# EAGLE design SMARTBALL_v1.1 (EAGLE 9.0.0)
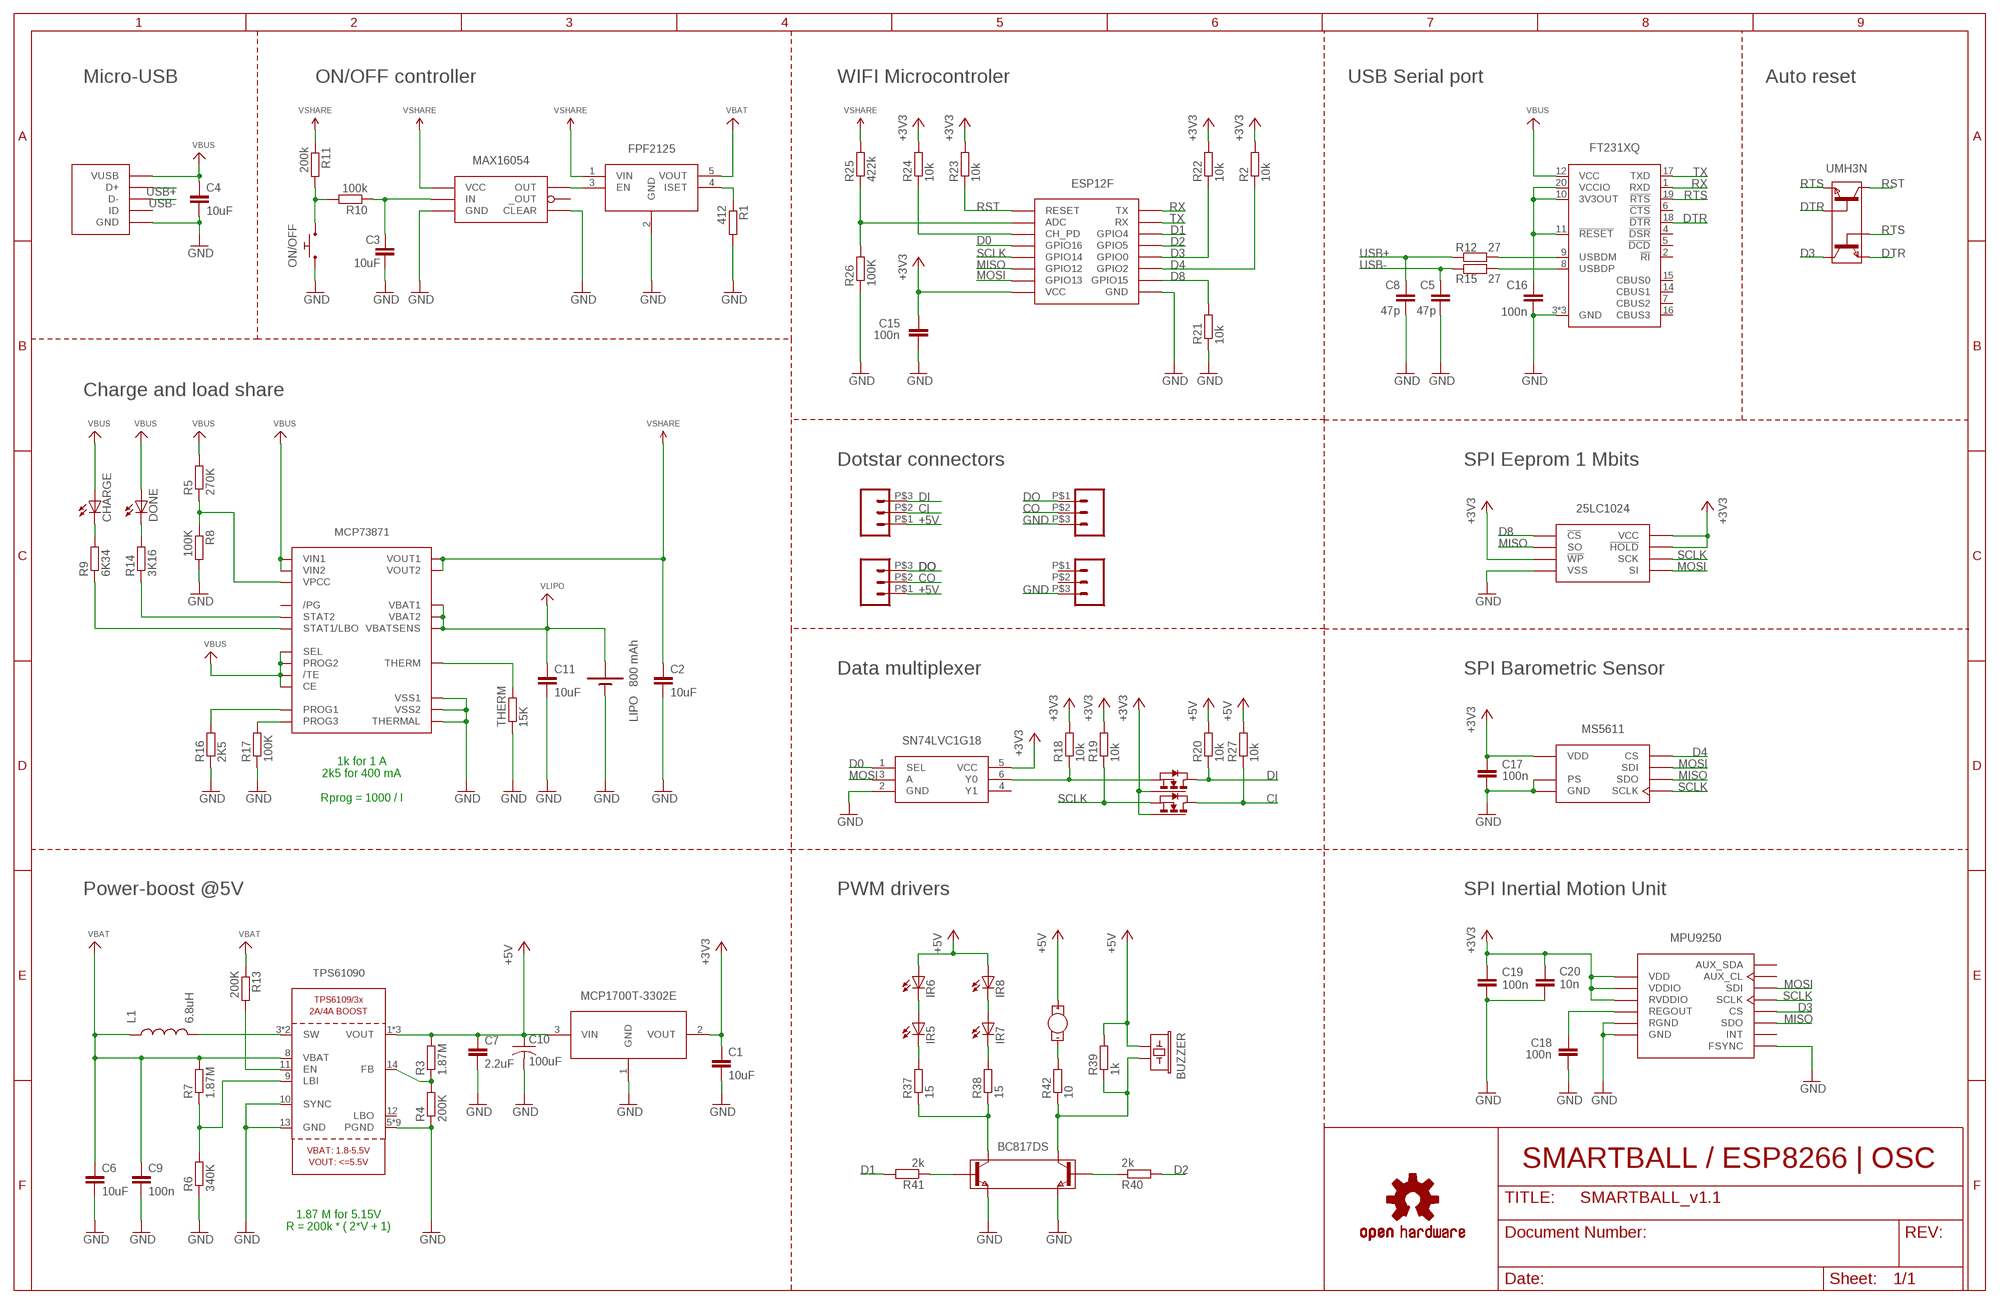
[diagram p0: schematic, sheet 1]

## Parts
BC817DS  BC817DS  [SOT457R_PHILIPS]
BUZZER  BUZZER_PKMCS0909E4000-R1  [BUZZER_PKMCS0909E4000-R1]
C1  10uF  C-EUC0603K  [C0603K]
C2  10uF  C-EUC0603K  [C0603K]
C3  10uF  C-EUC0603K  [C0603K]
C4  10uF  C-EUC0603K  [C0603K]
C5  47p  C-EUC0603K  [C0603K]
C6  10uF  C-EUC0603K  [C0603K]
C7  2.2uF  C-EUC0603K  [C0603K]
C8  47p  C-EUC0603K  [C0603K]
C9  100n  C-EUC0603K  [C0603K]
C10  100uF  C-USC1210  [C1210]
C11  10uF  C-EUC0603K  [C0603K]
C15  100n  C-EUC0603K  [C0603K]
C16  100n  C-EUC0603K  [C0603K]
C17  100n  C-EUC0603K  [C0603K]
C18  100n  C-EUC0603K  [C0603K]
C19  100n  C-EUC0603K  [C0603K]
C20  10n  C-EUC0603K  [C0603K]
CHARGE  KINGBRIGHT_16X08  [KINGBRIGHT_16X08]
DONE  KINGBRIGHT_16X08  [KINGBRIGHT_16X08]
ESP12F  ESP12  [ESP12]
FT231XQ  FT231X  [QFN20]
IR5  LED-SFH4050  [SFH4050]
IR6  LED-SFH4050  [SFH4050]
IR7  LED-SFH4050  [SFH4050]
IR8  LED-SFH4050  [SFH4050]
L1  6.8uH  ASPIAIG-S4035  [ASPIAIG-S4035]
LIPO  BATTERY_CONNECTOR  [MOTOR_CONNECTOR]
LOGO1  OSHW-LOGOL  [OSHW-LOGO-L]
MCP73871  MCP73871  [QFN20_4MM]
MOTOR  MOTOR_CONNECTOR  [MOTOR_CONNECTOR]
ON/OFF  B3U-3000P-B  [B3U-3000P-B]
R1  412  R-EU_R0402  [R0402]
R2  10k  R-EU_R0402  [R0402]
R3  1.87M  R-EU_R0402  [R0402]
R4  200K  R-EU_R0402  [R0402]
R5  270K  R-EU_R0402  [R0402]
R6  340K  R-EU_R0402  [R0402]
R7  1.87M  R-EU_R0402  [R0402]
R8  100K  R-EU_R0402  [R0402]
R9  6K34  R-EU_R0402  [R0402]
R10  100k  R-EU_R0402  [R0402]
R11  200k  R-EU_R0402  [R0402]
R12  27  R-EU_R0402  [R0402]
R13  200K  R-EU_R0402  [R0402]
R14  3K16  R-EU_R0402  [R0402]
R15  27  R-EU_R0402  [R0402]
R16  2K5  R-EU_R0402  [R0402]
R17  100K  R-EU_R0402  [R0402]
R18  10k  R-EU_R0402  [R0402]
R19  10k  R-EU_R0402  [R0402]
R20  10k  R-EU_R0402  [R0402]
R21  10k  R-EU_R0402  [R0402]
R22  10k  R-EU_R0402  [R0402]
R23  10k  R-EU_R0402  [R0402]
R24  10k  R-EU_R0402  [R0402]
R25  422k  R-EU_R0402  [R0402]
R26  100K  R-EU_R0402  [R0402]
R27  10k  R-EU_R0402  [R0402]
R37  15  R-EU_R0402  [R0402]
R38  15  R-EU_R0402  [R0402]
R39  1k  R-EU_R0402  [R0402]
R40  2k  R-EU_R0402  [R0402]
R41  2k  R-EU_R0402  [R0402]
R42  10  R-EU_R0402  [R0402]
THERM  15K  R-EU_R0402  [R0402]
TPS61090  TPS61090RSAR  VREG_TPS6103X  [PVQFN-16]
U$1  MOLEX-USB  [MOLEX-USB]
U$2  FPF2125  [SOT23-5]
U$3  MCP1700T  [SOT23-3]
U$5  CONN_03_SMD  [CONN03_SMD]
U$6  CONN_03_SMD  [CONN03_SMD]
U$12  MAX16054  [TSOT23-6]
U$14  CONN_03_SMD  [CONN03_SMD]
U$15  CONN_03_SMD  [CONN03_SMD]
U$16  25LC1024DFN-S  [DFN-S]
U$17  MS5611  [MS5611-QFN]
U$20  SN74LVC1G18  [DCK_R-PDSO-G6]
U$21  MPU-9250QFN24G  [QFN24G-0.4-3X3MM]
U$22  2N7002PS  [SOT363_PHILIPS]
UMH3N  UMH3N  [SOT363_PHILIPS]

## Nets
+3V3 [+3v3]: C1.1 C15.1 C17.1 C19.1 C20.2 ESP12F.VCC R2.2 R18.2 R19.2 R22.2 R23.2 R24.2 U$3.2(VOUT) U$16.3(!WP) U$16.7(!HOLD) U$16.8(VCC) U$17.P$1(VDD) U$20.5(VCC) U$21.1(RVDDIO) U$21.8(VDDIO) U$21.13(VDD) U$22.2(G1) U$22.5(G2)
+5V [power]: BUZZER.P$1 C7.1 C10.1 IR6.P$1(A) IR8.P$1(A) MOTOR.+ R3.2 R20.2 R27.2 R39.2 TPS61090.1(VOUT) TPS61090.15(VOUT) TPS61090.16(VOUT) U$3.3(VIN) U$5.P$1 U$15.P$1
CI: R27.1 U$5.P$2 U$22.3(D2)
CO: U$6.P$2 U$15.P$2
D0: ESP12F.GPIO16 U$20.1(SEL)
D1: ESP12F.GPIO4 R41.2
D2: ESP12F.GPIO5 R40.2
D3: ESP12F.GPIO0 R22.1 U$21.22(CS) UMH3N.3(C2)
D4: ESP12F.GPIO2 R2.1 U$17.P$4(CS) U$17.P$5(CS)
D8: ESP12F.GPIO15 R21.2 U$16.1(!CS)
DI: R20.1 U$5.P$3 U$22.6(D1)
DO: U$6.P$1 U$15.P$3
DTR: FT231XQ.18(!DTR) UMH3N.2(B1) UMH3N.4(E2)
EN1: ESP12F.CH_PD R24.1
ENABLE: R13.2 TPS61090.11(EN)
GND [power]: BC817DS.1(E1) BC817DS.4(E2) C1.2 C2.2 C3.2 C4.2 C5.2 C6.2 C7.2 C8.2 C9.2 C10.2 C11.2 C15.2 C16.2 C17.2 C18.2 C19.2 C20.1 ESP12F.GND FT231XQ.3(GND) FT231XQ.13(GND) FT231XQ.EXP(GND) LIPO.- MCP73871.P$10(VSS1) MCP73871.P$11(VSS2) MCP73871.P$21(THERMAL) ON/OFF.P$1 R1.2 R4.1 R6.1 R8.2 R16.1 R17.1 R21.1 R26.1 THERM.1 TPS61090.5(PGND) TPS61090.6(PGND) TPS61090.7(PGND) TPS61090.10(SYNC) TPS61090.13(GND) TPS61090.P$18(PGND) TPS61090.P$19(PGND) TPS61090.P$20(PGND) TPS61090.P$21(PGND) TPS61090.P$22(PGND) TPS61090.THERMAL(PGND) U$1.GND U$1.P$1(GND) U$1.P$11(GND) U$1.SHELL1(GND) U$1.SHELL2(GND) U$1.SHELL5(GND) U$1.SHELL6(GND) U$2.2(GND) U$3.1(GND) U$6.P$3 U$12.CLEAR U$12.GND U$14.P$3 U$16.4(VSS) U$17.P$2(PS) U$17.P$3(GND) U$20.2(GND) U$21.11(FSYNC) U$21.18(GND) U$21.20(RGND)
MISO: ESP12F.GPIO12 U$16.2(SO) U$17.P$6(SDO) U$21.9(SDO)
MOSI: ESP12F.GPIO13 U$16.5(SI) U$17.P$7(SDI) U$20.3(A) U$21.24(SDI)
N$1: U$2.3(EN) U$12.OUT
N$2: R1.1 U$2.4(ISET)
N$3: MCP73871.P$2(VPCC) R5.1 R8.1
N$4: MCP73871.P$13(PROG1) R16.2
N$5: FT231XQ.9(USBDM) R12.2
N$6: FT231XQ.8(USBDP) R15.2
N$8: ON/OFF.P$2 R10.2 R11.2
N$9: C3.1 R10.1 U$12.IN
N$11: R18.1 U$20.6(Y0) U$22.1(S1)
N$12: ESP12F.ADC R25.1 R26.2
N$17: L1.P$2 TPS61090.3(SW) TPS61090.4(SW)
N$18: R6.2 R7.1 TPS61090.9(LBI)
N$21: R3.1 R4.2 TPS61090.14(FB)
N$22: MCP73871.P$7(STAT2) R14.1
N$23: MCP73871.P$8(STAT1/LBO) R9.1
N$25: MCP73871.P$5(THERM) THERM.2
N$26: DONE.CATHODE(C) R14.2
N$27: CHARGE.CATHODE(C) R9.2
N$28: MCP73871.P$12(PROG3) R17.2
N$55: IR5.P$2(C) R37.2
N$56: IR5.P$1(A) IR6.P$2(C)
N$57: BC817DS.3(C2) R37.1 R38.1
N$58: IR7.P$2(C) R38.2
N$59: IR7.P$1(A) IR8.P$2(C)
N$60: BC817DS.6(C1) BUZZER.P$2 R39.1 R42.1
N$61: MOTOR.- R42.2
N$62: BC817DS.5(B2) R41.1
N$63: BC817DS.2(B1) R40.1
REGOUT1: C18.1 U$21.10(REGOUT)
RST: ESP12F.RESET R23.1 UMH3N.6(C1)
RTS: FT231XQ.19(!RTS) UMH3N.1(E1) UMH3N.5(B2)
RX: ESP12F.TX FT231XQ.1(RXD)
SCLK: ESP12F.GPIO14 R19.1 U$16.6(SCK) U$17.P$8(SCLK) U$21.23(SCLK) U$22.4(S2)
TX: ESP12F.RX FT231XQ.17(TXD)
USB+: C8.1 R12.1 U$1.D+
USB-: C5.1 R15.1 U$1.D-
VBAT [power]: C6.1 C9.1 L1.P$1 R7.2 R13.1 TPS61090.8(VBAT) U$2.5(VOUT)
VBUS [power]: C4.1 CHARGE.ANODE(A) DONE.ANODE(A) FT231XQ.12(VCC) MCP73871.P$3(SEL) MCP73871.P$4(PROG2) MCP73871.P$9(/TE) MCP73871.P$17(CE) MCP73871.P$18(VIN1) MCP73871.P$19(VIN2) R5.2 U$1.VUSB
VCCIO1: C16.1 FT231XQ.10(3V3OUT) FT231XQ.11(!RESET) FT231XQ.20(VCCIO)
VLIPO: C11.1 LIPO.+ MCP73871.P$14(VBAT1) MCP73871.P$15(VBAT2) MCP73871.P$16(VBATSENS)
VSHARE [power]: C2.1 MCP73871.P$1(VOUT1) MCP73871.P$20(VOUT2) R11.1 R25.2 U$2.1(VIN) U$12.VCC
Unconnected: FT231XQ.2(!RI) FT231XQ.4(!DSR) FT231XQ.5(!DCD) FT231XQ.6(!CTS) FT231XQ.7(CBUS2) FT231XQ.14(CBUS1) FT231XQ.15(CBUS0) FT231XQ.16(CBUS3) MCP73871.P$6(/PG) TPS61090.12(LBO) U$1.ID U$12._OUT U$14.P$1 U$14.P$2 U$20.4(Y1) U$21.7(AUX_CL) U$21.12(INT) U$21.21(AUX_SDA)

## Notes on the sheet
- Micro-USB | ON/OFF controller | WIFI Microcontroler | USB Serial port | Auto reset
- FPF2125
- MAX16054
- Charge and load share
- Dotstar connectors | SPI Eeprom 1 Mbits
- Data multiplexer | SPI Barometric Sensor
- 800 mAh
- SN74LVC1G18
- 1k for 1 A
  2k5 for 400 mA
  
  Rprog = 1000 / I
- Power-boost @5V | PWM drivers | SPI Inertial Motion Unit
- MCP1700T-3302E
- SMARTBALL / ESP8266 | OSC
- 1.87 M for 5.15V
  R = 200k * ( 2*V + 1)

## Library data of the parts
BC817DS = Smartball:BC817DS
BUZZER = Smartball:BUZZER_PKMCS0909E4000-R1
C1-C9 C11 C15-C20 = rcl:C-EU: CAPACITOR, European symbol; SPICEPREFIX: C
C10 = rcl:C-US: CAPACITOR, American symbol
CHARGE DONE = Smartball:KINGBRIGHT_16X08
ESP12F = esp8266modules:ESP12: ESP8266 Wifi module 12
FT231XQ = Smartball:FT231X
IR5-IR8 = Smartball:LED-SFH4050: 850 nm High Power IR Led from OSRAM
L1 = Smartball:ASPIAIG-S4035
LIPO = Smartball:BATTERY_CONNECTOR
LOGO1 = SparkFun-Aesthetics:OSHW-LOGO: Open-Source Hardware (OSHW) Logo
MCP73871 = microbuilder:MCP73871: MCP73871 Lithium Polymer Battery Charger Digikey: MCP73871-2CCI/ML-ND
MOTOR = Smartball:MOTOR_CONNECTOR
ON/OFF = Smartball:B3U-3000P-B
R1-R27 R37-R42 THERM = rcl:R-EU_: RESISTOR, European symbol; SPICEPREFIX: R
TPS61090 = microbuilder:VREG_TPS6103X: TPS6103x 4A Boost - 1.8-5.5V Input, Adjustable Output to 5.5V
U$1 = Smartball:MOLEX-USB
U$2 = Smartball:FPF2125
U$3 = Smartball:MCP1700T
U$5 U$6 U$14 U$15 = Smartball:CONN_03_SMD
U$12 = Smartball:MAX16054
U$16 = Smartball:25LC1024: Microship 25LC1024 1Mbit SPI EEPROM
U$17 = Smartball:MS5611: MS5611 barometric sensor
U$20 = Smartball:SN74LVC1G18
U$21 = Smartball:MPU-9250: MPU-9250 Invensense IMU Chipset
U$22 = Smartball:2N7002PS
UMH3N = Smartball:UMH3N

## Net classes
0 default: width 0.152 mm
1 power: width 0.254 mm
2 +3v3: width 0.203 mm

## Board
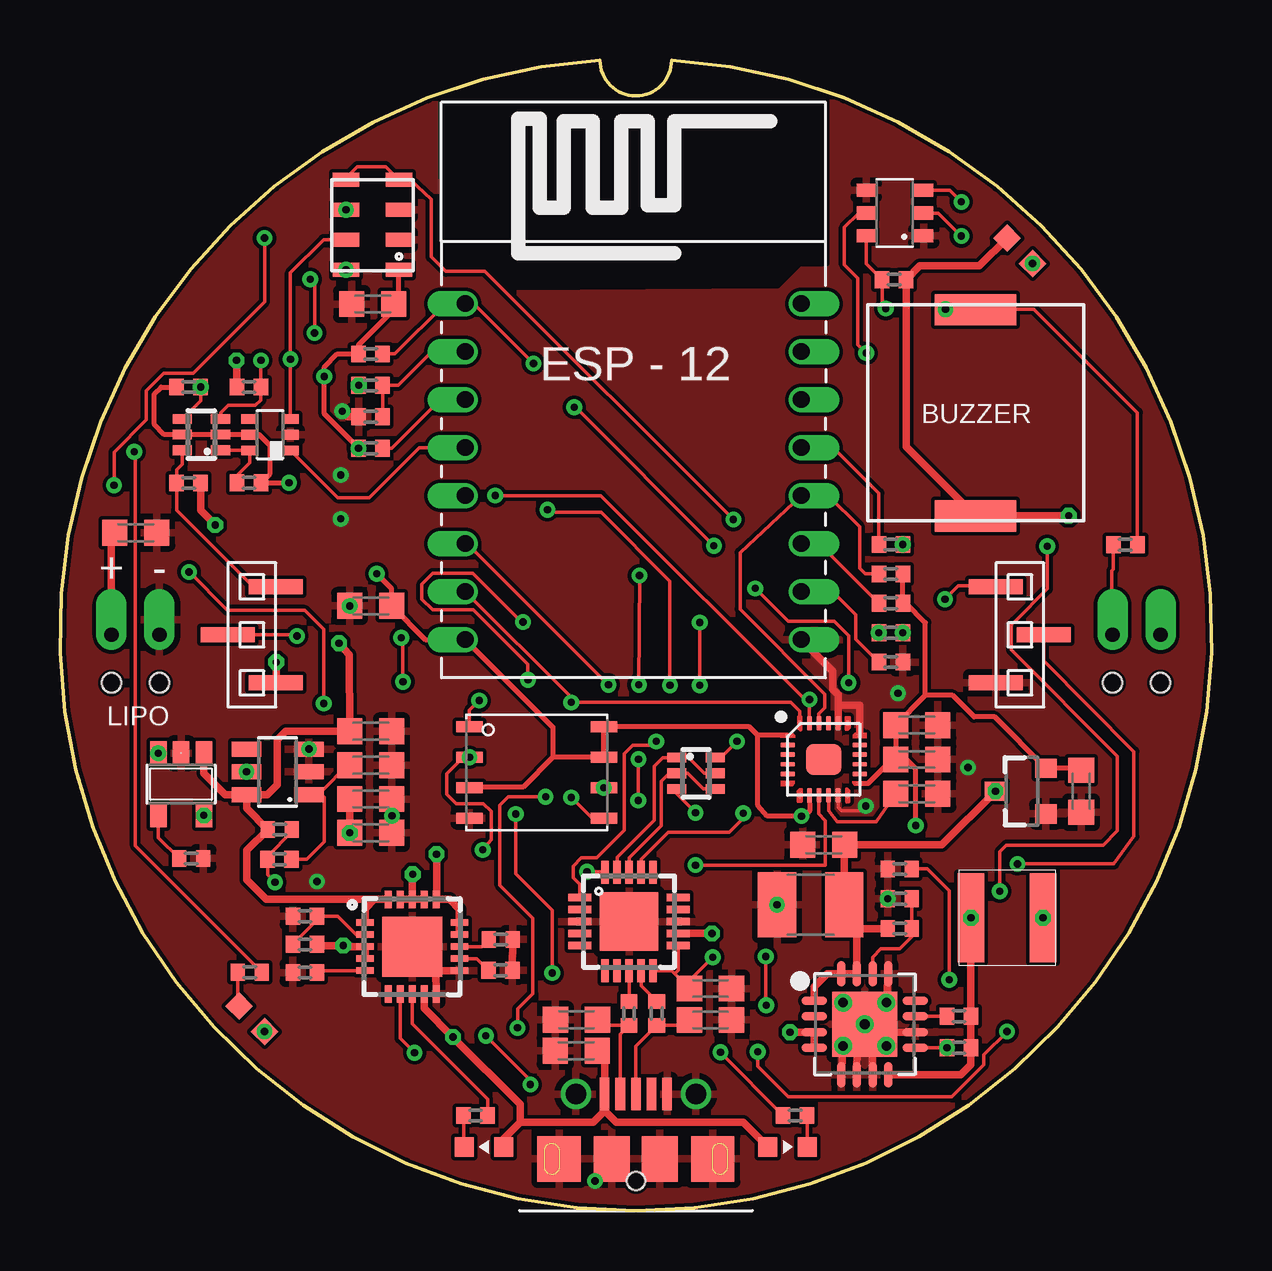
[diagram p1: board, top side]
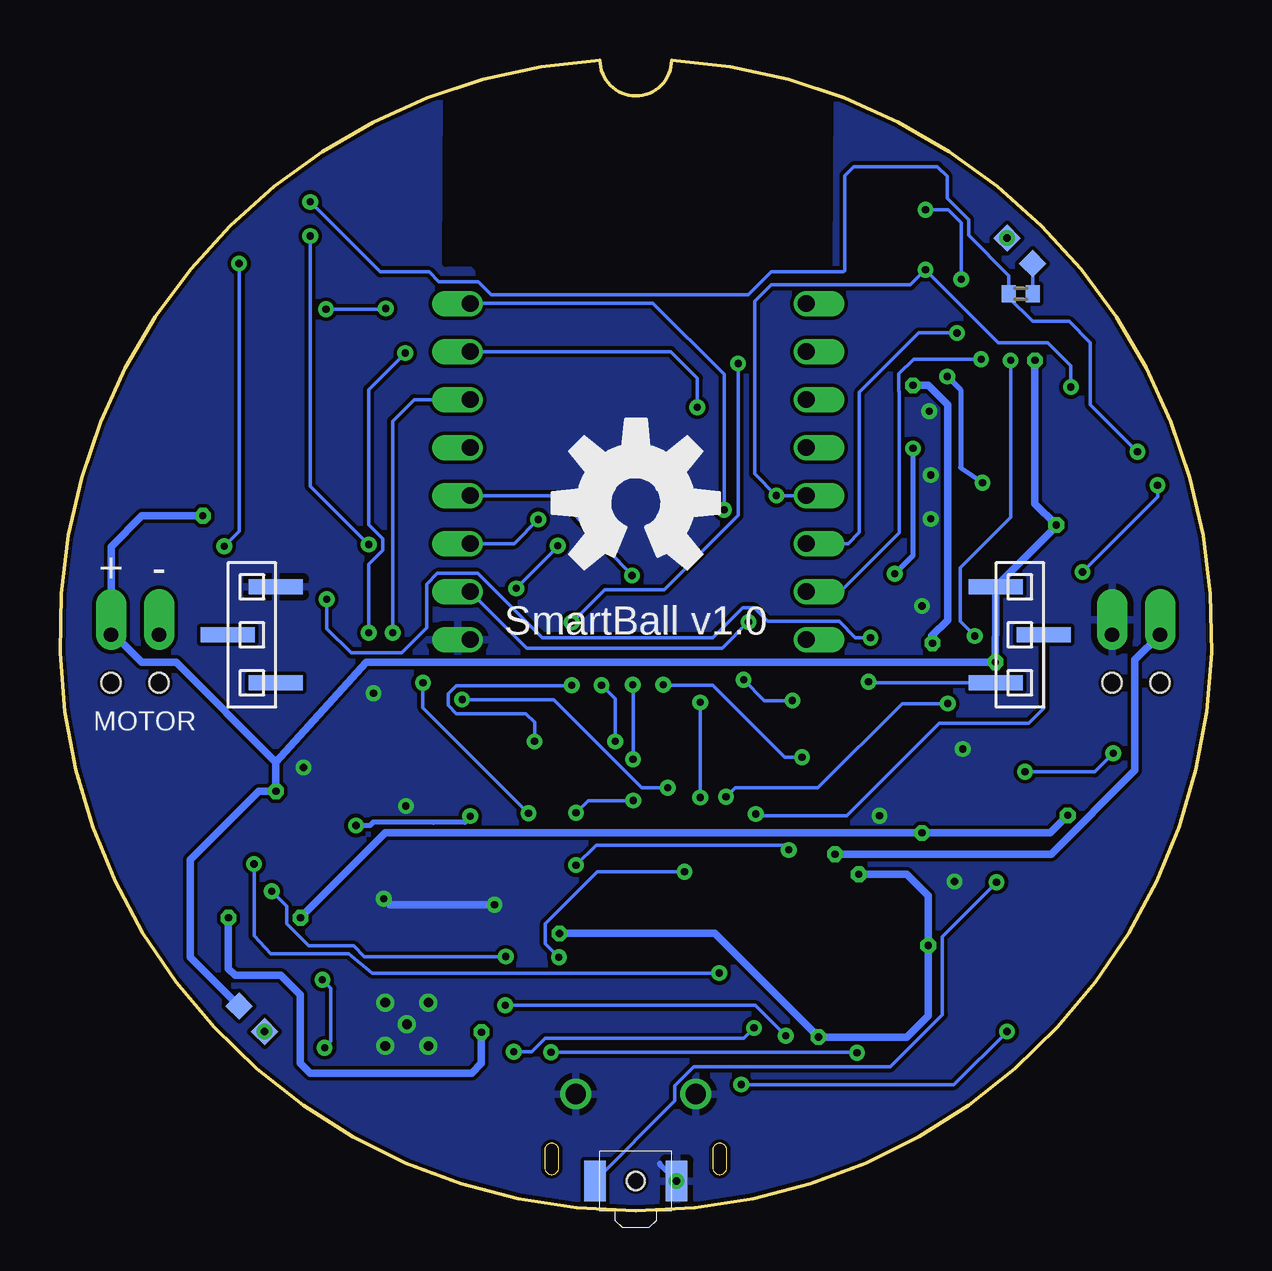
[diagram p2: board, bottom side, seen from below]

Size 47.98 x 47.96 mm. Coordinates in mm from the lower left corner, seen from the top.
Outline: 22.5,47.96 arc353 25.49,47.96 arc-180 22.5,47.96
Copper layers (1*16): Top 0.035mm / dielectric 1.5mm / Bottom 0.035mm
Design rules "PCBWay-LIMIT": minimum track width 4mil, minimum drill 0.3mm, track to track 6mil, track to pad 6mil, pad to pad 6mil, via to via 6mil, smd to smd 6mil, copper to edge 6mil, drill to drill 6mil, minimum pad ring 7mil, minimum via ring 7mil, stop-mask expansion 4mil, vias tented up to drill 25mil, thermal gap 10mil

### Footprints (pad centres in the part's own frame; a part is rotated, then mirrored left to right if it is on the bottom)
SOT457R_PHILIPS = smd 0.55 x 0.8: 1 -0.95,-1.2; 2 0,-1.2; 3 0.95,-1.2; 4 0.95,1.2; 5 0,1.2; 6 -0.95,1.2
BUZZER_PKMCS0909E4000-R1 = smd 1.3 x 3.4: P$1 -4.3,0; P$2 4.3,0
C0603K = smd 1.05 x 1.08: 1 -0.875,0; 2 0.875,0
C1210 = smd 1.6 x 2.7: 1 -1.4,0; 2 1.4,0
KINGBRIGHT_16X08 = smd 0.8 x 0.8: ANODE 0,0; CATHODE 1.65,0
ESP12 = drill 0.7 offset: ADC -7.1,3.8; CH_PD -7.1,1.8; GND 6.9,-8.2; GPIO0 6.9,-2.2; GPIO2 6.9,-4.2; GPIO4 6.9,1.8; GPIO5 6.9,-0.2; GPIO12 -7.1,-4.2; GPIO13 -7.1,-6.2; GPIO14 -7.1,-2.2; GPIO15 6.9,-6.2; GPIO16 -7.1,-0.2; RESET -7.1,5.8; RX 6.9,3.8; TX 6.9,5.8; VCC -7.1,-8.2
QFN20 = smd 0.95 x 0.3: 1 -2.05,1; 2 -2.05,0.5; 3 -2.05,0; 4 -2.05,-0.5; 5 -2.05,-1; 11 2.05,-1; 12 2.05,-0.5; 13 2.05,0; 14 2.05,0.5; 15 2.05,1 | smd 0.3 x 0.95: 6 -1,-2.05; 7 -0.5,-2.05; 8 0,-2.05; 9 0.5,-2.05; 10 1,-2.05; 16 1,2.05; 17 0.5,2.05; 18 0,2.05; 19 -0.5,2.05; 20 -1,2.05 | smd 2.45 x 2.45: EXP 0,0
SFH4050 = smd 0.8 x 0.8: P$1 -0.75,0; P$2 0.75,0
ASPIAIG-S4035 = smd 1.1 x 3.7: P$1 -1.5,0; P$2 1.5,0
MOTOR_CONNECTOR = drill 0.6 pad 1.27 offset: + 0,0; - 2,0 | hole 0.8: 0,-2; 2,-2
QFN20_4MM = smd 0.73 x 0.28: P$1 -1.965,1; P$2 -1.965,0.5; P$3 -1.965,0; P$4 -1.965,-0.5; P$5 -1.965,-1; P$11 1.965,-1; P$12 1.965,-0.5; P$13 1.965,0; P$14 1.965,0.5; P$15 1.965,1 | smd 0.28 x 0.73: P$6 -1,-1.965; P$7 -0.5,-1.965; P$8 0,-1.965; P$9 0.5,-1.965; P$10 1,-1.965; P$16 1,1.965; P$17 0.5,1.965; P$18 0,1.965; P$19 -0.5,1.965; P$20 -1,1.965 | smd 2.5 x 2.5: P$21 0,0
B3U-3000P-B = smd 0.9 x 1.7: P$1 0,0; P$2 3.4,0 | hole 0.75: 1.7,0
R0402 = smd 0.6 x 0.7: 1 -0.5,0; 2 0.5,0
PVQFN-16 = smd 1.05 x 0.35: 1 -2.1,0.975; 2 -2.1,0.325; 3 -2.1,-0.325; 4 -2.1,-0.975; 9 2.1,-0.975; 10 2.1,-0.325; 11 2.1,0.325; 12 2.1,0.975 | smd 0.35 x 1.05: 5 -0.975,-2.1; 6 -0.325,-2.1; 7 0.325,-2.1; 8 0.975,-2.1; 13 0.975,2.1; 14 0.325,2.1; 15 -0.325,2.1; 16 -0.975,2.1 | drill 0.4: P$18 0,0; P$19 -0.9,0.9; P$20 0.9,0.9; P$21 0.9,-0.9; P$22 -0.9,-0.9 | smd 2.7 x 2.7: THERMAL 0,0
MOLEX-USB = smd 0.4 x 1.35: D+ 0,2.7; D- -0.65,2.7; GND 1.3,2.7; ID 0.65,2.7; VUSB -1.3,2.7 | smd 1.8 x 1.9: P$1 -3.2,0; P$11 3.2,0 | drill 0.85: SHELL1 -2.5,2.7; SHELL2 2.5,2.7 | smd 1.5 x 1.9: SHELL5 -1,0; SHELL6 1,0
SOT23-5 = smd 0.69 x 0.99: 1 -0.95,-1.29; 2 0,-1.29; 3 0.95,-1.29; 4 0.95,1.3; 5 -0.95,1.3
SOT23-3 = smd 0.8 x 0.9: 1 -0.95,-1; 2 0.95,-1; 3 0,1.1
CONN03_SMD = smd 0.635 x 2.25: P$1 -2,-1; P$2 0,1; P$3 2,-1
TSOT23-6 = smd 0.62 x 1.22: _OUT 0.95,1.3; CLEAR 0.95,-1.3; GND 0,-1.3; IN -0.95,-1.3; OUT 0,1.3; VCC -0.95,1.3
DFN-S = smd 1.1 x 0.45: 1 -2.8,1.905; 2 -2.8,0.635; 3 -2.8,-0.635; 4 -2.8,-1.905; 5 2.8,-1.905; 6 2.8,-0.635; 7 2.8,0.635; 8 2.8,1.905
MS5611-QFN = smd 1.1 x 0.6: P$1 -2.2,3.75; P$2 -2.2,2.5; P$3 -2.2,1.25; P$4 -2.2,0; P$5 0,0; P$6 0,1.25; P$7 0,2.5; P$8 0,3.75
DCK_R-PDSO-G6 = smd 0.4 x 0.7: 1 -0.65,-0.85; 2 0,-0.85; 3 0.65,-0.85; 4 0.65,0.85; 5 0,0.85; 6 -0.65,0.85
QFN24G-0.4-3X3MM = smd 0.2 x 0.15: 1 -1.5,1; 6 -1.5,-1; 13 1.5,-1; 18 1.5,1 | smd 0.6 x 0.2: 2 -1.5,0.6; 3 -1.5,0.2; 4 -1.5,-0.2; 5 -1.5,-0.6; 14 1.5,-0.6; 15 1.5,-0.2; 16 1.5,0.2; 17 1.5,0.6 | smd 0.15 x 0.2: 7 -1,-1.5; 12 1,-1.5; 19 1,1.5; 24 -1,1.5 | smd 0.2 x 0.6: 8 -0.6,-1.5; 9 -0.2,-1.5; 10 0.2,-1.5; 11 0.6,-1.5; 20 0.6,1.5; 21 0.2,1.5; 22 -0.2,1.5; 23 -0.6,1.5 | smd 1.5 x 1.3: 25 0,0
SOT363_PHILIPS = smd 0.4 x 0.8: 1 -0.65,-0.8; 2 0,-0.8; 3 0.65,-0.8; 4 0.65,0.8; 5 0,0.8; 6 -0.65,0.8

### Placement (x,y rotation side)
BC817DS  34.79,41.58 90 top
BUZZER  38.15,33.26 90 top
C1  42.55,17.49 270 top
C2  12.94,19.99 0 top
C3  12.94,18.58 0 top
C4  21.51,6.67 180 top
C5  21.52,7.97 180 top
C6  12.94,15.76 0 top
C7  31.82,15.26 180 top
C8  27.1,7.96 0 top
C9  12.94,17.17 0 top
C10  31.28,12.76 180 top
C11  3.15,28.26 0 top
C15  12.94,25.21 180 top
C16  27.11,9.27 0 top
C17  13.03,37.79 180 top
C18  35.7,17.38 0 top
C19  35.7,18.81 0 top
C20  35.7,20.25 180 top
CHARGE  18.49,2.67 180 top
DONE  29.49,2.67 0 top
ESP12F  23.99,32.01 0 top
FT231XQ  23.71,12.06 0 top
IR5  7.99,8.01 135 top
IR6  39.99,40.01 315 top
IR7  7.99,40.01 315 bottom
IR8  39.99,8.01 315 bottom
L1  39.46,12.21 0 top
LIPO  2.14,24.01 0 top
LOGO1  23.99,29.51 0 bottom
MCP73871  14.67,11.02 0 top
MOTOR  45.86,24.01 0 bottom
ON/OFF  22.29,1.25 180 bottom
R1  5.47,14.69 0 top
R2  34.62,25.32 0 top
R3  34.99,11.77 180 top
R4  34.99,13.01 0 top
R5  10.2,11.11 0 top
R6  34.99,14.25 0 top
R7  37.46,6.8 0 top
R8  10.2,12.28 180 top
R9  17.31,3.98 180 top
R10  9.15,14.65 180 top
R11  9.16,15.89 0 top
R12  24.86,8.23 90 top
R13  37.46,8.11 180 top
R14  30.63,3.98 0 top
R15  23.71,8.23 90 top
R16  18.36,11.31 180 top
R17  18.35,10.03 180 top
R18  7.87,30.34 0 top
R19  5.36,34.33 180 top
R20  5.36,30.33 0 top
R21  34.62,22.87 180 top
R22  34.62,26.54 0 top
R23  12.94,35.71 180 top
R24  12.94,31.78 180 top
R25  12.94,34.4 180 top
R26  12.94,33.09 0 top
R27  7.87,34.33 180 top
R37  7.9,9.95 180 top
R38  7.95,38.22 0 bottom
R39  34.76,38.81 0 top
R40  34.62,27.77 180 top
R41  34.62,24.1 180 top
R42  44.39,27.76 180 top
THERM  10.2,9.94 0 top
TPS61090  33.53,7.78 0 top
U$1  23.99,2.17 0 top
U$2  5.05,17.78 180 top
U$3  40.08,17.49 90 top
U$5  7.99,24.01 90 top
U$6  39.99,24.01 270 top
U$12  9.07,18.3 90 top
U$14  39.99,24.01 90 bottom
U$15  7.99,24.01 270 bottom
U$16  19.86,18.27 0 top
U$17  11.92,42.97 180 top
U$20  8.75,32.34 90 top
U$21  31.82,18.81 0 top
U$22  5.89,32.35 90 top
UMH3N  26.5,18.24 270 top

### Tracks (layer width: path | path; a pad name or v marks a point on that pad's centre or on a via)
+3V3  (via drill 0.3)
  Top 0.203: C1.1 42.47,18.44 U$3.2 38.94,20.58 38.09,20.58 37.19,21.48 36.06,21.48 | C19.1 C20.2 36.06,21.48 | U$21.13 33.67,17.81 34.67,18.81 C19.1 | 36.06,21.48 36.06,24.52 35.26,25.32 R2.2 R22.2 | U$21.8 31.23,16.67 31.01,16.45 v30.89,16.45 29.47,16.45 29.07,16.9 29.07,19.81 29.08,19.81 | U$21.1 29.08,19.81 | 29.08,19.81 28.72,20.17 U$16.8 U$16.7 20.54,18.9 | 20.54,18.9 19.29,17.66 17.09,17.66 U$16.3 | 20.54,18.9 20.54,20.16 ESP12F.VCC 15.22,23.81 C15.1 13.82,25.93 v13.2,26.55 | R24.2 11.01,33.21 v11.01,34.77 11.01,35.16 11.56,35.71 R23.2 12.44,36.08 13.9,37.54 C17.1 14.12,38.01 U$17.P$1 | v9.54,30.34 R18.2 8.75,30.72 8.75,31.89 8.3,32.34 U$20.5 U$22.2 U$22.5 4.35,32.35 3.93,32.78 3.93,34.05 4.21,34.33 R19.2 | v35.65,16.06 35.65,18.42 35.26,18.81 C19.1
  Bottom 0.203: v30.89,16.45 31.11,16.19 32.43,16.19 34.93,16.2 35.07,16.06 v35.65,16.06 | v11.01,34.77 10.46,34.21 10.46,30.97 v9.54,30.34 | v13.2,26.55 12.44,27.31 R24.2
  other vias: 12.44,31.78
+5V  (via drill 0.3)
  Top 0.305: 33.21,11.69 TPS61090.15 TPS61090.16 31.96,9.88 31.43,9.35 TPS61090.1 | 33.21,11.69 33.21,12.23 C10.1 32.68,15.24 C7.1 36.75,15.26 U$3.3 | R3.2 33.28,11.77 33.21,11.69 | v42.03,28.97 BUZZER.P$1 35.26,31.85 R39.2 35.83,39.38 38.3,39.38 IR6.P$1 | v9.01,22.87 9.02,21.98 U$5.P$1 | v6.47,28.58 5.86,29.19 R20.2 | v7.36,35.44 7.37,35.43 R27.2
  Bottom 0.305: MOTOR.+ 45.85,24.14 | 45.85,24.14 45.85,27.68 44.57,28.97 v42.03,28.97 | v7.36,35.44 7.36,29.47 v6.47,28.58 6.47,28.53 U$15.P$1 8.99,25.05 v9.01,22.87 35.23,22.87 38.98,18.71 | 38.98,18.71 U$3.3 39.71,17.49 42.56,14.64 42.56,10.58 IR8.P$1 | 38.98,18.71 43.15,22.87 44.58,22.87 45.85,24.14
  other vias: 38.98,17.49
CI  (via drill 0.3)
  Top 0.152: U$22.3 6.69,33.25 7,33.56 8.14,33.56 8.37,33.79 R27.1 v8.37,35.44 | v9.87,23.96 9.82,24.01 U$5.P$2
  Bottom 0.152: v8.37,35.44 8.37,28.91 10.48,26.81 10.48,24.57 v9.87,23.96
CO  (via drill 0.3)
  Top 0.152: v18.99,16.54 18.99,14.06 20.51,12.53 v20.51,9.92 | v39.89,14.46 43.91,14.46 44.75,15.61 44.75,19.14 40.99,22.92 U$6.P$2
  Bottom 0.152: U$15.P$2 6.99,20.95 7.61,20.33 11.34,20.33 15.21,16.47 18.91,16.47 v18.99,16.54 | v20.51,9.92 34.97,9.92 35.96,10.73 39.21,10.73 39.89,11.46 v39.89,14.46
D0
  Top 0.152: 9.62,31.68 U$20.1 11.57,29.73 12.89,29.73 14.98,31.81 ESP12F.GPIO16
D1  (via drill 0.3)
  Bottom 0.152: R41.2 34.12,32.91 33.22,33.81 ESP12F.GPIO4
  other vias: 34.12,24.1
D2
  Top 0.152: R40.2 34.12,29.92 32.22,31.81 ESP12F.GPIO5
D3  (via drill 0.3)
  Top 0.152: R22.1 33.55,26.54 33.32,26.78 33.32,28.51 32.01,29.81 ESP12F.GPIO0 28.34,27.43 28.34,25.08 31.87,21.52 31.87,20.96 31.62,20.72 U$21.22 | v24.12,21.93 v24.15,26.48 | v24.1,18.82 24.1,17.11 v24.1,17.1 | v26.48,16.6 25.7,17.38 UMH3N.3
  Bottom 0.152: v24.1,18.82 24.1,21.91 v24.12,21.93 | v24.15,26.48 27.28,29.81 ESP12F.GPIO0 | v24.1,17.1 25.97,17.1 v26.48,16.6
D4  (via drill 0.3)
  Top 0.152: R2.1 31.63,27.81 ESP12F.GPIO2 | v28.06,28.81 17.69,39.15 16.07,39.15 15.46,39.76 15.46,42.15 14.59,42.97 U$17.P$4 13.57,43.52 12.39,43.52 11.92,43.05 U$17.P$5
  Bottom 0.152: ESP12F.GPIO2 29.06,27.81 v28.06,28.81
D8  (via drill 0.3)
  Top 0.152: R21.2 33.16,23.83 33.16,24.85 32.2,25.81 ESP12F.GPIO15 | U$16.1 17.06,20.86 v17.47,21.27 | v19.29,24.55 19.5,24.34 19.43,24.34 17.2,26.57 15.52,26.57 15.08,26.12 15.08,25.5 15.52,25.05 17.22,25.05 19.5,22.77 v19.5,22.13
  Bottom 0.152: v17.47,21.27 18.63,21.27 v19.5,22.13 | v19.29,24.55 20.39,23.45 28.53,23.45 ESP12F.GPIO15
DI
  Top 0.152: U$22.6 5.1,31.12 4.86,30.89 R20.1 4.86,29.2 8.05,26.01 U$5.P$3
DO  (via drill 0.3)
  Top 0.152: v14.29,22.06 14.29,23.81 v14.21,23.89 | v36.87,25.49 37.43,26.04 38.96,26.04 U$6.P$1
  Bottom 0.152: U$15.P$3 14.24,22.01 v14.29,22.06 | v14.21,23.89 14.84,23.89 15.52,24.57 18.49,24.57 19.05,25.13 19.54,25.13 20.78,23.89 27.9,23.89 30.58,26.57 32.26,26.57 32.7,26.12 32.7,24.3 33.75,23.25 35.08,23.25 35.09,23.26 35.24,23.25 35.86,23.25 36.87,24.27 v36.87,25.49
DTR
  Top 0.152: UMH3N.4 26.81,17.59 26.16,18.24 UMH3N.2 25.38,18.24 25.06,17.92 25.06,16.06 23.71,14.71 FT231XQ.18
EN1
  Top 0.152: R24.1 13.83,31.78 15.87,33.82 ESP12F.CH_PD
ENABLE
  Top 0.152: TPS61090.11 R13.2
GND  (via drill 0.3)
  Top 0.152: U$21.18 | U$21.11 32.42,16.83 32.58,16.67 33.37,16.67 v33.57,16.88
  Top 0.203: U$1.SHELL5 22.99,1.95 ON/OFF.P$1
  Top 0.305: TPS61090.10 34.48,7.45 TPS61090.P$21 | TPS61090.13 TPS61090.P$20 | TPS61090.5 TPS61090.P$22 | TPS61090.6 33.21,6.84 33.49,7.66 | 33.49,7.66 TPS61090.THERMAL | TPS61090.7 33.82,6.77 33.49,7.66 | MCP73871.P$10 15.66,10.02 | 15.66,10.02 15.66,10.07 MCP73871.P$21 | MCP73871.P$11 15.66,10.02 | R17.1 R16.1 | R26.1 11.99,33.09 v11.76,33.32 | ESP12F.GND 32.2,22.5 32.2,21.73 32.43,21.51 32.43,21.02 | U$21.18 33.32,21.07 32.48,21.07 32.43,21.02 | U$21.20 32.43,21.02 | U$1.P$11 27.49,2.17 | U$1.P$1 20.49,2.17
  Bottom 0.203: ON/OFF.P$1 22.99,1.95 22.99,2.01
  Bottom 0.305: C10.2 34.24,12.76 R4.1
  other vias: 34.92,21.57 37.84,18.48 10.37,19.25 12.07,25.21 13.83,16.47 10.71,13.73 11.7,30.67 11.7,28.84 29.88,12.76 34.49,13.01 22.29,1.25
  pour Top: -0.01,0.01 47.99,0.01 47.99,48.01 -0.01,48.01
  pour Bottom: -0.01,48.01 -0.01,0.01 47.99,0.01 47.99,48.01
MISO  (via drill 0.3)
  Top 0.152: U$21.9 31.62,16.56 31.89,16.27 31.89,14.41 v26.48,14.41 | v22.85,21.93 16.97,27.81 ESP12F.GPIO12 | v10.61,36.59 10.61,38.64 v10.43,38.82 | v17.62,15.05 17.97,15.48 17.97,16.65 17.64,16.98 16.5,16.98 16.12,17.36 16.12,18.22 16.8,18.9 v17.06,18.9
  Bottom 0.152: v17.06,18.9 17.79,18.9 20.79,21.9 22.83,21.9 v22.85,21.93 | ESP12F.GPIO12 15.14,27.81 14.67,28.28 14.67,34.12 12.21,36.59 v10.61,36.59 | v10.43,38.82 10.43,41.18 10.97,41.72 U$17.P$6 | v26.48,14.41 25.64,15.25 17.59,15.25 v17.62,15.05
  other vias: 11.92,41.72
MOSI  (via drill 0.3)
  Top 0.152: U$20.3 v9.6,35.49 9.6,39.08 10.99,40.47 U$17.P$7 | ESP12F.GPIO13 21.3,21.4 v21.3,21.19 30.45,21.19 30.82,20.82 U$21.24 | v21.3,17.23 22.17,16.36 U$16.5
  Bottom 0.152: v21.3,21.19 v21.3,17.23 | ESP12F.GPIO13 15.47,25.81 13.02,28.25 13.02,34.16 13.02,34.88 12.41,35.49 v9.6,35.49
N$1  (via drill 0.3)
  Bottom 0.152: U$2.3 4.87,18.3 U$12.OUT
  other vias: 4.1,19.07 7.77,18.3
N$2
  Top 0.152: U$2.4 4.1,15.56 R1.1
N$3
  Top 0.152: R5.1 10.7,12.11 R8.1 11.57,12.28 12.34,11.52 MCP73871.P$2
N$4
  Top 0.152: MCP73871.P$13 17.57,11.02 R16.2
N$5
  Top 0.152: R12.2 24.21,9.38 FT231XQ.9
N$6
  Top 0.152: R15.2 FT231XQ.8
N$7
  cutout Bottom: 11.52,43.09 11.52,39.2 14.47,39.23 14.14,39.68 14.14,42.74 14.49,43.09
N$8  (via drill 0.3)
  Top 0.152: R11.2 9.66,15.8 8.65,14.79 R10.2 8.65,14.01 v8.96,13.7
  Bottom 0.152: ON/OFF.P$2 22.36,4.59 22.36,5.23 21.58,6.01 13.39,6.01 11.22,8.18 11.22,11.44 v8.96,13.7
N$9
  Top 0.152: R10.1 10.29,14.65 11.01,15.38 11.01,17.23 10.9,17.35 | 10.9,17.35 U$12.IN | C3.1 11.98,18.58 10.9,17.49 10.9,17.35
N$10
  cutout Top: 11.52,43.09 11.52,39.23 14.47,39.25 14.11,39.73 14.11,42.72 14.49,43.09
N$11
  Top 0.152: U$22.1 U$20.6 7.92,31.68 7.92,31.18 7.37,30.63 R18.1
N$12
  Top 0.152: ESP12F.ADC 16.88,35.82 15.51,35.82 14.09,34.4 R25.1 R26.2
N$13
  cutout Top: 15.93,46.53 15.96,39.44 18.04,39.44 18.91,38.52 29.89,38.59 30.8,39.51 31.9,39.49 31.9,46.58
N$14
  cutout Bottom: 15.91,46.55 15.96,39.44 17.99,39.44 18.91,38.52 29.89,38.62 30.78,39.51 31.9,39.49 31.87,46.58
N$17  (via drill 0.3)
  Top 0.305: v30.42,7.45 v30.42,7.46 TPS61090.3 TPS61090.4
  Bottom 0.305: v30.42,7.45 30.42,6.16 30.83,5.75 37.56,5.75 37.96,6.16 37.96,9 38.78,9.81 40.68,9.81 40.96,10.09 L1.P$2
  other vias: 40.96,12.21
N$18  (via drill 0.3)
  Top 0.152: TPS61090.9 R7.1 | v37.05,9.64 37.05,13.34 36.13,14.26 36.13,14.25 R6.2
  Bottom 0.152: R7.1 36.69,7.07 36.69,9.28 v37.05,9.64
  other vias: 36.96,6.8
N$21
  Top 0.152: TPS61090.14 33.86,10.58 34.2,10.93 34.99,10.93 35.49,11.43 R3.1 R4.2
N$22  (via drill 0.3)
  Top 0.152: R14.1 27.52,6.58 v27.52,6.61 | v14.77,6.59 14.17,7.19 MCP73871.P$7
  Bottom 0.152: v27.52,6.61 14.8,6.61 v14.77,6.59
N$23
  Top 0.152: R9.1 17.81,4.66 14.67,7.8 MCP73871.P$8
N$25
  Top 0.152: THERM.2 10.78,10.02 MCP73871.P$5
N$26
  Top 0.152: DONE.CATHODE 31.14,3.97 R14.2
N$27
  Top 0.152: R9.2 16.81,2.7 CHARGE.CATHODE
N$28
  Top 0.152: MCP73871.P$12 17.37,10.52 R17.2
N$55
  Top 0.152: R37.2 7.4,8.6 IR5.P$2
N$56  (via drill 0.3)
  Top 0.152: v41.14,27.7 41.14,25.92 39.78,24.56 39.77,24.56 39.64,24.42 39.64,23.38 44.06,18.96 44.06,15.83 43.48,15.25 39.44,15.25 39.16,14.97 v39.16,13.32 | v29.4,10.6 29.4,8.59 v29.43,8.57 | v17.75,7.3 19.6,5.45 v19.6,5.27
  Bottom 0.152: IR6.P$2 40.52,28.31 v41.14,27.7 | v39.16,13.32 38.54,12.71 38.54,11.97 37.61,11.04 35.75,11.04 35.3,10.6 v29.4,10.6 | v29.43,8.57 19.02,8.57 v17.75,7.3 | v19.6,5.27 10.73,5.27 IR5.P$1
  other vias: 40.52,39.48 8.52,7.48
N$57  (via drill 0.3)
  Top 0.152: BC817DS.3 37.07,42.53 v37.56,42.05 | R37.1 3.14,15.21 3.14,31.58 v3.09,31.63
  Bottom 0.152: v37.56,42.05 34.64,39.13 32.6,39.13 32.2,38.72 30.55,38.72 30.01,38.19 19.29,38.19 18.35,39.13 15.34,39.13 15.28,39.18 15.28,43.14 14.9,43.52 11.42,43.52 11.01,43.11 11.01,42.2 10.13,41.31 10.13,40.65 8.45,38.97 R38.1 8.45,38.06 7.46,37.07 5.93,37.07 5.05,36.18 5.05,33.59 v3.09,31.63
N$58
  Bottom 0.152: R38.2 IR7.P$2
N$59  (via drill 0.3)
  Top 0.152: IR8.P$2 38.48,6.5 38.48,6.09 37.16,4.76 30.34,4.76 29.07,6.03 v29.07,6.64 | v19.07,7.63 19.07,8.42 19.7,9.05 19.7,12.2 18.33,13.57 18.33,16.9 18.68,17.26 v20.23,17.26 | v10.99,21.14 10.99,24.24 10.2,25.03 6.98,25.03 v5.38,26.63 | v2.25,30.24 2.25,31.62 3.6,32.96 3.6,34.18 4.32,34.91 5.54,34.91 8.52,37.89 IR7.P$1
  Bottom 0.152: v29.07,6.64 28.32,6.64 27.76,7.19 19.5,7.19 v19.07,7.63 | v20.23,17.26 19.85,17.64 16.4,17.64 12.89,21.14 v10.99,21.14 | v5.38,26.63 2.25,29.75 v2.25,30.24
  other vias: 39.46,7.48 8.52,40.54
N$60  (via drill 0.3)
  Top 0.152: BC817DS.6 33.59,39.47 R39.1 34.26,37.75 v34.41,37.6 | R42.1 44.89,33.27 40.58,37.58 38.17,37.58 BUZZER.P$2 36.92,37.56 v36.9,37.58
  Bottom 0.152: v36.9,37.58 34.43,37.58 v34.41,37.6
N$61
  Top 0.152: R42.2 43.89,26.74 43.83,26.68 43.83,24.03 MOTOR.-
N$62  (via drill 0.3)
  Top 0.152: v33.59,35.75 33.24,36.1 33.24,38.87 32.68,39.43 32.68,40.98 33.28,41.58 BC817DS.5
  Bottom 0.152: v33.59,35.75 35.12,34.22 35.12,28.59 34.54,28.01 34.54,27.53 35.12,26.95 R41.1
  other vias: 35.12,24.1
N$63  (via drill 0.3)
  Top 0.152: v37.56,40.62 36.6,41.58 BC817DS.2
  Bottom 0.152: R40.1 37.56,30.21 v37.56,40.62
  other vias: 35.12,27.77
REGOUT1
  Top 0.152: U$21.10 32.02,16.67 32.38,16.21 34.01,16.21 C18.1
RST  (via drill 0.3)
  Top 0.152: R23.1 13.95,35.71 16.05,37.81 ESP12F.RESET 17.23,37.81 v19.73,35.32 | UMH3N.6 27.53,18.89 v28.21,19.57 | v26.66,21.9 v26.66,24.52
  Bottom 0.152: v28.21,19.57 28.21,20.35 28.58,20.73 31.47,20.73 31.81,21.07 31.81,21.55 31.47,21.89 26.67,21.89 v26.66,21.9 | v26.66,24.52 25.29,25.89 22.81,25.89 19.73,28.98 v19.73,35.32
RTS
  Top 0.152: UMH3N.5 26.85,18.24 26.2,18.89 UMH3N.1 25.12,18.89 24.76,18.53 24.76,16.29 23.21,14.75 FT231XQ.19
RX  (via drill 0.3)
  Top 0.152: FT231XQ.1 21.66,13.61 21.38,13.89 21.38,14.37 21.72,14.71 22.37,14.71 23.51,15.86 23.51,19.06 23.86,19.4 24.68,19.4 v24.85,19.57 | v25.42,21.9 25.42,26.25 22.55,29.12 20.41,29.12 v20.31,29.22
  Bottom 0.152: v24.85,19.57 24.85,21.34 v25.42,21.9 | v20.31,29.22 20.31,34.86 23.28,37.83 30.87,37.83 ESP12F.TX
SCLK  (via drill 0.3)
  Top 0.152: U$22.4 5.86,33.77 R19.1 | v18.13,29.81 22.54,29.81 31.22,21.13 | U$21.23 31.22,21.13 | 31.22,21.13 v31.23,21.31
  Bottom 0.152: ESP12F.GPIO14 v18.13,29.81 19.04,30.72 19.04,37.91 18.35,38.59 12.55,38.59 U$17.P$8 8.88,36.18 6.82,36.18 5.86,35.22 R19.1 | v31.23,21.31 27.41,21.31 23.74,17.64 U$16.6
  other vias: 11.92,39.22 5.86,34.33 22.66,17.63
TX  (via drill 0.3)
  Top 0.152: FT231XQ.17 24.21,14.65 25.34,15.78 27.88,15.78 28.46,16.37 v28.46,16.57 | v28.97,25.94 30.35,24.57 32.26,24.57 32.86,23.97 v32.86,22.01 | v27.24,27.72 21.48,33.49 v21.43,33.49
  Bottom 0.152: v28.46,16.57 32.86,20.96 v32.86,22.01 | v28.97,25.94 27.24,27.67 v27.24,27.72 | v21.43,33.49 21.43,34.71 22.53,35.81 ESP12F.RX
USB+
  Top 0.152: U$1.D+ 23.99,6.86 R12.1 26,7.73 C8.1
USB-
  Top 0.152: U$1.D- 23.34,7.36 R15.1 22.64,7.73 C5.1
VBAT  (via drill 0.3)
  Top 0.305: C6.1 C9.1 | TPS61090.8 37.54,5.68 37.96,6.1 R7.2 R13.1 L1.P$1
  Bottom 0.305: U$2.5 6.72,15.76 C6.1 34.42,15.76 L1.P$1
  other vias: 6,16.48 12.07,15.76 37.96,12.21
VBUS  (via drill 0.3)
  Top 0.254: 10.8,11.02 R5.2
  Top 0.305: C4.1 22.69,6.37 U$1.VUSB 22.69,4.17 | 22.69,4.17 22.22,3.69 19.17,3.69 | 19.17,3.69 18.49,3.02 CHARGE.ANODE | DONE.ANODE 28.47,3.69 23.17,3.69 22.69,4.17 | MCP73871.P$9 15.17,8.45 v16.37,7.25 19.17,4.45 19.17,3.69 | MCP73871.P$4 MCP73871.P$3 11.84,11.02 v11.8,11.06 10.75,11.06 R5.2 | MCP73871.P$19 MCP73871.P$18 | MCP73871.P$18 MCP73871.P$17 | MCP73871.P$18 14.67,14.01 v14.7,14.03 | v27.17,11.57 FT231XQ.12
  Bottom 0.305: v14.7,14.03 12.69,14.03 11.8,13.14 v11.8,11.06 11.8,8.14 12.69,7.25 v16.37,7.25 20.69,11.57 v27.17,11.57
VCCIO1  (via drill 0.3)
  Top 0.152: 25.62,9.89 C16.1 26.23,9.61 v27.19,10.58 | 25.62,9.89 25.49,10.01 FT231XQ.10 | FT231XQ.11 25.76,10.03 25.62,9.89 | v21.96,14.13 22.69,14.13 FT231XQ.20
  Bottom 0.152: v27.19,10.58 27.75,11.13 27.75,11.97 25.59,14.13 v21.96,14.13
VLIPO  (via drill 0.3)
  Top 0.305: MCP73871.P$14 MCP73871.P$15 16.64,12.57 16.23,12.98 MCP73871.P$16 15.69,12.99 v15.69,14.87 | LIPO.+ 2.14,28.12 C11.1
  Bottom 0.305: LIPO.+ 3.19,22.96 3.19,18.36 6.68,14.87 v15.69,14.87
VSHARE  (via drill 0.3, 0.3 pad 0.4)
  Top 0.305: U$12.VCC 6.88,17.35 5.98,18.25 6,18.26 U$2.1 | U$12.VCC 7.77,16.78 R11.1 7.79,15.02 7.79,13.8 8.6,12.99 13.1,12.99 | MCP73871.P$1 12.71,12.6 13.1,12.99 | 13.1,12.99 13.11,12.98 MCP73871.P$20 | U$12.VCC 8.64,17.35 9.06,17.76 9.06,19.64 9.4,19.99 C2.1 12.06,23.17 v11.62,23.66
  Bottom 0.305: v11.62,23.66 11.65,23.96 10.99,24.62 10.99,33.59 11.8,34.4 R25.2
  other vias: 12.44,34.4

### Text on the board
tPlace: BUZZER | LIPO
bPlace: SmartBall v1.0 | MOTOR

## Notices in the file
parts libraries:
microbuilder: This work is placed in the public domain, and may be freely used for commercial and non-commercial work with the following conditions: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
SparkFun-Aesthetics: Licensing: Creative Commons ShareAlike 4.0 International - https://creativecommons.org/licenses/by-sa/4.0
